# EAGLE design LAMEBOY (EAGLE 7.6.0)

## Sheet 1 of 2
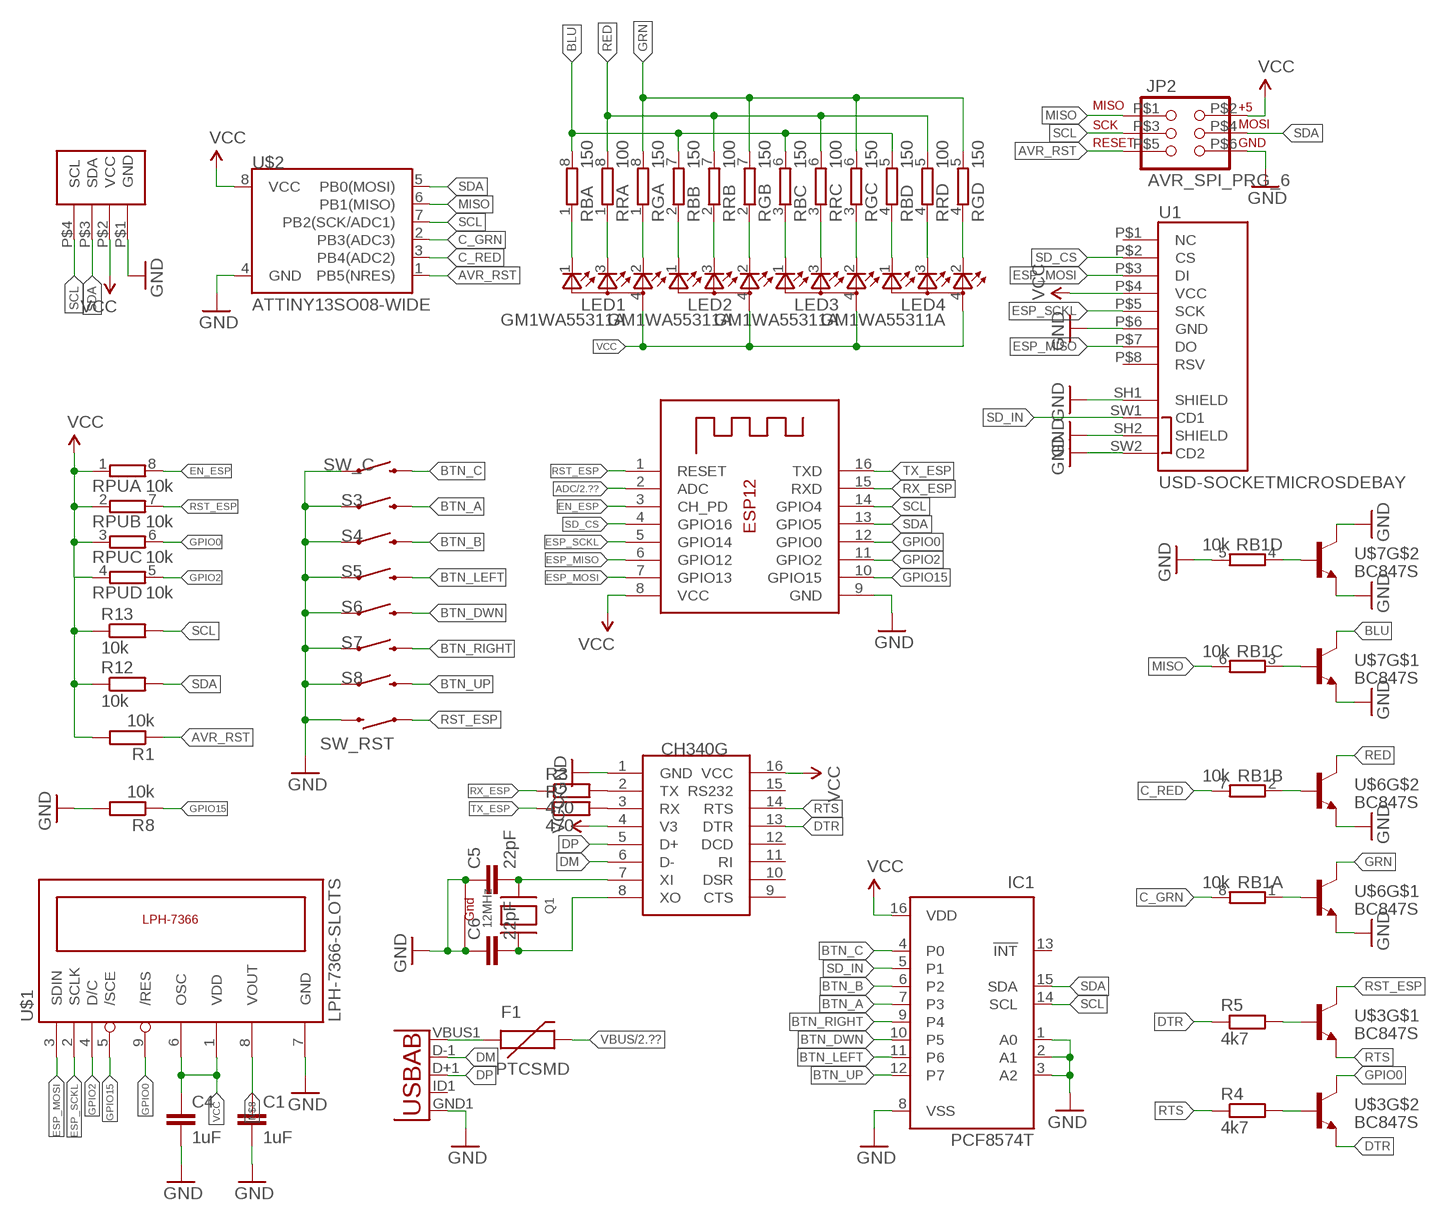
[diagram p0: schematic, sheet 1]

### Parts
C1  1uF  C-EUC0603K  [C0603K]
C4  1uF  C-EUC0603K  [C0603K]
C5  22pF  C-EUC0603K  [C0603K]
C6  22pF  C-EUC0603K  [C0603K]
CH340G  CH340GCH340G  [SOIC16]
F1  PTCSMD  [PTC-1206]
IC1  PCF8574T  [SO16W]
JP2  AVR_SPI_PRG_6  [2X3_SMD_PAD]
LED1  GM1WA55311A  [GM1WA55311A]
LED2  GM1WA55311A  [GM1WA55311A]
LED3  GM1WA55311A  [GM1WA55311A]
LED4  GM1WA55311A  [GM1WA55311A]
Q1  12MHz  XTAL-4-3225  [NX3225]
R1  10k  R-EU_R0603  [R0603]
R2  470  R-EU_R0603  [R0603]
R3  470  R-EU_R0603  [R0603]
R4  4k7  R-EU_R0603  [R0603]
R5  4k7  R-EU_R0603  [R0603]
R8  10k  R-EU_R0603  [R0603]
R12  10k  R-EU_R0603  [R0603]
R13  10k  R-EU_R0603  [R0603]
RB  150  4R-N0603-ARC  [0603-ARC]
RB1  10k  4R-N0603-ARC  [0603-ARC]
RG  150  4R-N0603-ARC  [0603-ARC]
RPU  10k  4R-N0603-ARC  [0603-ARC]
RR  100  4R-N0603-ARC  [0603-ARC]
S3  SWITCH-MOMENTARY-2SMD-4  [TACTILE_SWITCH_TALL]
S4  SWITCH-MOMENTARY-2SMD-4  [TACTILE_SWITCH_TALL]
S5  SWITCH-MOMENTARY-2SMD-4  [TACTILE_SWITCH_TALL]
S6  SWITCH-MOMENTARY-2SMD-4  [TACTILE_SWITCH_TALL]
S7  SWITCH-MOMENTARY-2SMD-4  [TACTILE_SWITCH_TALL]
S8  SWITCH-MOMENTARY-2SMD-4  [TACTILE_SWITCH_TALL]
SW_C  SWITCH-MOMENTARY-2-SMD-1101NE  [TACTILE-SWITCH-1101NE]
SW_RST  SWITCH-MOMENTARY-2-SMD-1101NE  [TACTILE-SWITCH-1101NE]
U1  USD-SOCKETMICROSDEBAY  [MICRO-SD-SOCKET-EBAY]
U2  USB  USB-ABCONN-11794  [USB-AB-MICRO-SMD_V03]
U$1  LPH-7366-SLOTS  [LPH-7366-SLOTS]
U$2  ATTINY13SO08-WIDE  [SO08-EIAJ]
U$3  BC847S  MMDT3904  [SOT363]
U$6  BC847S  MMDT3904  [SOT363]
U$7  BC847S  MMDT3904  [SOT363]
U$10  I2C_GROVE  [I2C_GROVE]
X1  ESP-12  [ESP-12]

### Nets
ADC: X1.2(ADC) ; also sheet 2
AVR_RST: JP2.P$5 R1.1 U$2.1(PB5(NRES))
BLU: RB.5 RB.6 RB.7 RB.8 U$7.3(C)
BTN_A: IC1.7(P3) S3.B2
BTN_B: IC1.6(P2) S4.B2
BTN_C: IC1.4(P0) SW_C.P$2
BTN_DWN: IC1.10(P5) S6.B2
BTN_LEFT: IC1.11(P6) S5.B2
BTN_RIGHT: IC1.9(P4) S7.B2
BTN_UP: IC1.12(P7) S8.B2
C_GRN: RB1.8 U$2.2(PB3(ADC3))
C_RED: RB1.7 U$2.3(PB4(ADC2))
DM: CH340G.6(D-) U2.D-1(D-)
DP: CH340G.5(D+) U2.D+1(D+)
DTR: CH340G.13(DTR) R5.1 U$3.1(E)
EN_ESP: RPU.8 X1.3(CH_PD)
ESP_MISO: U1.P$7(DO) X1.6(GPIO12)
ESP_MOSI: U1.P$3(DI) U$1.3(SDIN) X1.7(GPIO13)
ESP_SCKL: U1.P$5(SCK) U$1.2(SCLK) X1.5(GPIO14)
GND: C1.2 C4.2 C5.1 C6.1 CH340G.1(GND) IC1.1(A0) IC1.2(A1) IC1.3(A2) IC1.8(VSS) JP2.P$6 Q1.2(G2) Q1.4(G1) R8.2 RB1.5 S3.A2 S4.A2 S5.A2 S6.A2 S7.A2 S8.A2 SW_C.P$1 SW_RST.P$2 U1.P$6(GND) U1.SH1(SHIELD) U1.SH2(SHIELD) U1.SW2(CD2) U2.GND1(GND) U$1.7(GND) U$2.4(GND) U$6.1(E) U$6.4(E) U$7.1(E) U$7.4(E) U$7.6(C) U$10.P$1(GND) X1.9(GND) ; also sheet 2
GPIO0: RPU.6 U$1.9(/RES) U$3.6(C) X1.12(GPIO0)
GPIO2: RPU.5 U$1.4(D/C) X1.11(GPIO2)
GPIO15: R8.1 U$1.5(/SCE) X1.10(GPIO15)
GRN: RG.5 RG.6 RG.7 RG.8 U$6.3(C)
L2_R: LED1.3(CBLUE) RR.1
L3_B: LED1.1(CGREEN) RB.1
L4_G: LED1.2(CRED) RG.1
MISO: JP2.P$1 RB1.6 U$2.6(PB1(MISO))
N$1: LED4.1(CGREEN) RB.4
N$2: LED4.3(CBLUE) RR.4
N$3: LED4.2(CRED) RG.4
N$4: LED3.1(CGREEN) RB.3
N$5: LED3.3(CBLUE) RR.3
N$6: LED3.2(CRED) RG.3
N$7: LED2.1(CGREEN) RB.2
N$8: C1.1 U$1.8(VOUT)
N$9: LED2.3(CBLUE) RR.2
N$10: LED2.2(CRED) RG.2
N$11: RB1.1 U$6.5(B)
N$13: RB1.2 U$6.2(B)
N$17: C5.2 CH340G.7(XI) Q1.1(X1)
N$18: RB1.3 U$7.5(B)
N$19: RB1.4 U$7.2(B)
N$24: C6.2 CH340G.8(XO) Q1.3(X2)
N$25: R5.2 U$3.5(B)
N$26: CH340G.3(RX) R2.2
N$27: CH340G.2(TX) R3.2
N$28: R4.2 U$3.2(B)
RED: RR.5 RR.6 RR.7 RR.8 U$6.6(C)
RST_ESP: RPU.7 SW_RST.P$1 U$3.3(C) X1.1(RESET)
RTS: CH340G.14(RTS) R4.1 U$3.4(E)
RX_ESP: R3.1 X1.15(RXD)
SCL: IC1.14(SCL) JP2.P$3 R13.2 U$2.7(PB2(SCK/ADC1)) U$10.P$4(SCL) X1.14(GPIO4)
SD_CS: U1.P$2(CS) X1.4(GPIO16)
SD_IN: IC1.5(P1) U1.SW1(CD1)
SDA: IC1.15(SDA) JP2.P$4 R12.2 U$2.5(PB0(MOSI)) U$10.P$3(SDA) X1.13(GPIO5)
TX_ESP: R2.1 X1.16(TXD)
VBUS: F1.2 ; also sheet 2
VCC: C4.1 CH340G.4(V3) CH340G.16(VCC) IC1.16(VDD) JP2.P$2 LED1.4(A) LED2.4(A) LED3.4(A) LED4.4(A) R1.2 R12.1 R13.1 RPU.1 RPU.2 RPU.3 RPU.4 U1.P$4(VCC) U$1.1(VDD) U$1.6(OSC) U$2.8(VCC) U$10.P$2(VCC) X1.8(VCC) ; also sheet 2
VUSB: F1.1 U2.VBUS1(VBUS)
Unconnected: CH340G.9(CTS) CH340G.10(DSR) CH340G.11(RI) CH340G.12(DCD) CH340G.15(RS232) IC1.13(!INT) U1.P$1(NC) U1.P$8(RSV) U2.ID1(USBID)

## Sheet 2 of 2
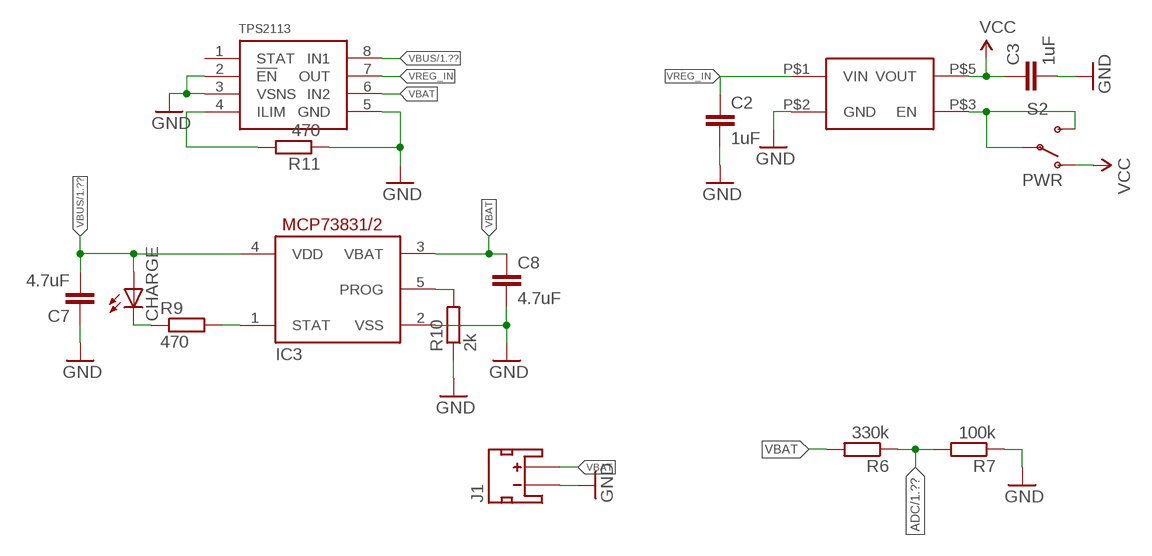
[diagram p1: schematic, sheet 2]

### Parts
C2  1uF  C-EUC0603K  [C0603K]
C3  1uF  C-EUC0603K  [C0603K]
C7  4.7uF  C-EUC0603K  [C0603K]
C8  4.7uF  C-EUC0603K  [C0603K]
CHARGE  LEDCHIP-LED0805  [CHIP-LED0805]
IC3  MCP73831  MCP73831/OT  [SOT23-5L]
J1  JST_2MM_MALE  [JST-2-SMD]
R6  330k  R-EU_R0603  [R0603]
R7  100k  R-EU_R0603  [R0603]
R9  470  R-EU_R0603  [R0603]
R10  2k  R-EU_R0603  [R0603]
R11  470  R-EU_R0603  [R0603]
S2  PWR  SWITCH-SPDT-SMD-A  [SWITCH-SPST-SMD-A]
U$4  TPS2113-PW  [TEXAS-PW]
U$9  AP2112KAP2112K  [AP2112]

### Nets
ADC: R6.1 R7.2 ; also sheet 1
GND: C2.2 C3.2 C7.1 C8.2 IC3.2(VSS) J1.1(-) R7.1 R10.1 R11.1 U$4.2(!EN) U$4.3(VSNS) U$4.5(GND) U$9.P$2(GND) ; also sheet 1
N$12: IC3.1(STAT) R9.2
N$15: CHARGE.C R9.1
N$20: R11.2 U$4.4(ILIM)
N$21: IC3.5(PROG) R10.2
VBAT: C8.1 IC3.3(VBAT) J1.2(+) R6.2 U$4.6(IN2)
VBUS: C7.2 CHARGE.A IC3.4(VDD) U$4.8(IN1) ; also sheet 1
VCC: C3.1 S2.1(O) U$9.P$5(VOUT) ; also sheet 1
VREG_IN: C2.1 U$4.7(OUT) U$9.P$1(VIN)
VREG_OUT: S2.2(P) S2.3(S) U$9.P$3(EN)
Unconnected: J1.NC1(PAD1) J1.NC2(PAD2) U$4.1(STAT)

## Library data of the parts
C1-C8 = rcl:C-EU: CAPACITOR, European symbol
CH340G = ch340g:CH340G: USB to TTL RS232 converter
CHARGE = led:LED: LED
F1 = SparkFun-PowerIC:PTC: Resettable Fuse PTC; PROD_ID: RES-11150
IC1 = micro-philips:PCF8574: I2C-Bus Remote 8-bit I/O expander http://www.semiconductors.philips.com/acrobat_download/datasheets/PCF8574_4.pdf; MPN: PCF8574T/3,512; OC_FARNELL: 1201255; OC_NEWARK: 70R6870
IC3 = adafruit:MCP73831: MCP73831/2 Miniature Single-Cell, Fully Integrated Li-Ion, Li-Polymer Charge Management Controllers. Nice and small simple lipoly charge controller, with adjustable current and status output (LED) http://www.ladyada.net/library/pcb/eaglelibrary.html
J1 = SparkFun-Connectors:JST_2MM_MALE: Mates to single-cell LiPo batteries. CONN-08352; PROD_ID: CONN-08352
JP2 = SparkFun-Connectors:AVR_SPI_PRG_6: AVR ISP 6 Pin This is the reduced ISP connector for AVR programming. Common on Arduino. This footprint will take up less PCB space and can be used with a 10-pin to 6-pin adapter such as SKU: BOB-08508 **Special note about "TEST_POINT" package. The stop mask is on the top side, so if you want your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
LED1-LED4 = led:GM1WA55311A: Chip LED RGB Source: http://document.sharpsma.com/files/GM1WA55311A_SS.pdf
Q1 = adafruit:XTAL-4: Classic 4-pin 3.2 x 2.5mm crystal
R1-R13 = rcl:R-EU_: RESISTOR, European symbol
RB RB1 RG RPU RR = resistor-dil:4R-N: Array Chip Resistor Source: RS Component / Phycomp; OC_FARNELL: unknown; OC_NEWARK: unknown
S2 = SparkFun-Electromechanical:SWITCH-SPDT: SPDT Switch Simple slide switch, Spark Fun Electronics SKU : COM-00102 DPDT SMT slide switch, AYZ0202, SWCH-08179
S3-S8 = SparkFun-Electromechanical:SWITCH-MOMENTARY-2: Various NO switches- pushbuttons, reed, etc; PROD_ID: SWCH-11966
SW_C SW_RST = SparkFun-Electromechanical:SWITCH-MOMENTARY-2: Various NO switches- pushbuttons, reed, etc
U1 = SparkFun-Connectors:USD-SOCKET: microSD Socket Push-push type uSD socket. Schematic element and footprint production proven. Spark Fun Electronics SKU : PRT-00127. tDoc lines correctly indicate media card edge positions when inserting (unlocked, locked, depressed). NOTE: CD1 and CD2 are connected internally
U2 = SparkFun-Connectors:USB-AB: This is a USB AB connector that is compatible with USB OTG. i.e. this connector can serve as a host or device; PROD_ID: CONN-11794
U$1 = lph-7366:LPH-7366-SLOTS
U$2 = SparkFun-DigitalIC:ATTINY13: Atmel 8-pin 1kB flash uC
U$3 U$6 U$7 = SparkFun-DiscreteSemi:MMDT3904: Dual NPN transistor
U$4 = TPS2113:TPS2113-PW
U$9 = TPS2113:AP2112K
U$10 = TPS2113:I2C_GROVE
X1 = adafruit:ESP-12

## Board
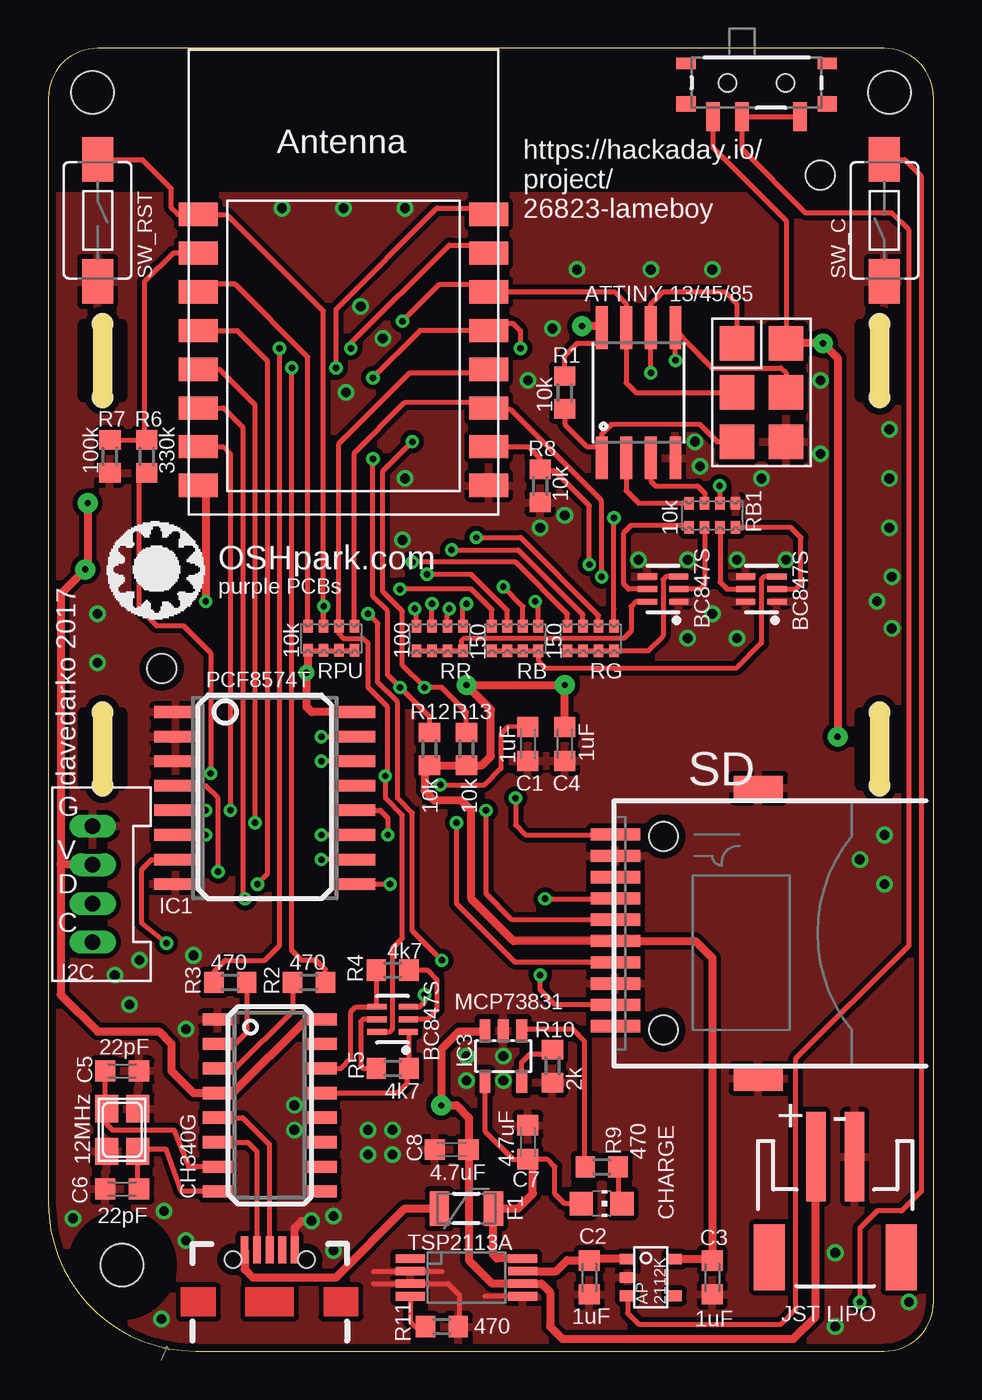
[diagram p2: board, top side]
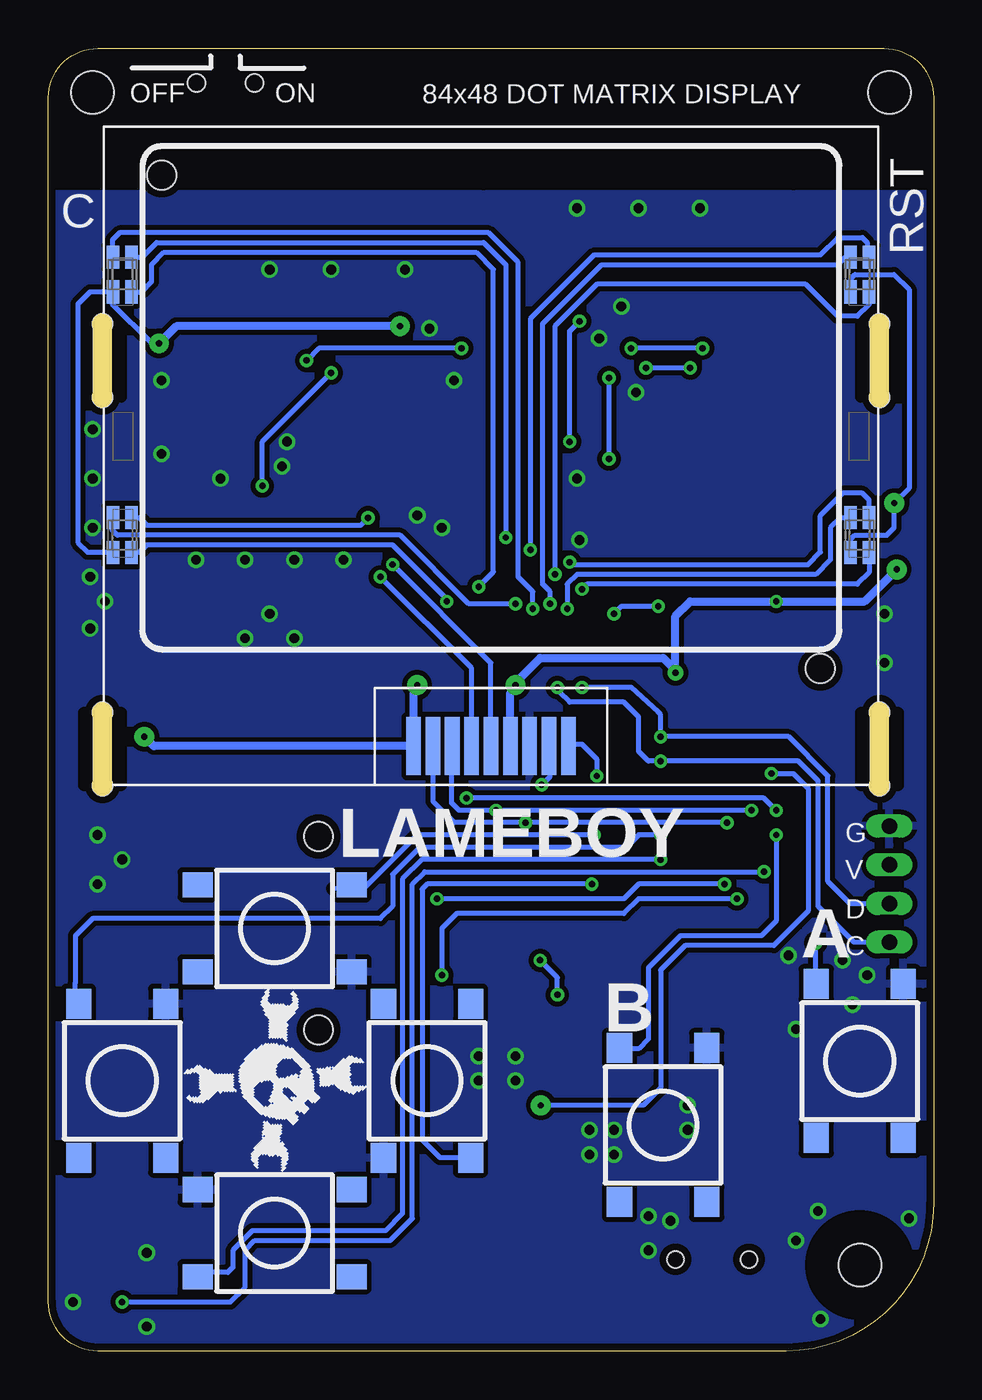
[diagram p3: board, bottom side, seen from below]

Size 45.72 x 67.31 mm. Coordinates in mm from the lower left corner, seen from the top.
Outline: 0,64.77 0,7.62 arc90 7.62,0 43.18,0 arc90 45.72,2.54 45.72,64.77 arc90 43.18,67.31 2.54,67.31 arc90 0,64.77
Copper layers (1*16): Top 0.0356mm / dielectric 1.5011mm / Bottom 0.0356mm
Design rules "LaenPCBOrder *": minimum track width 6mil, minimum drill 13mil, track to track 6mil, track to pad 6mil, pad to pad 6mil, via to via 6mil, smd to smd 6mil, copper to edge 15mil, drill to drill 6mil, minimum pad ring 7mil, minimum via ring 7mil, stop-mask expansion 3mil, vias tented up to drill 200mil, thermal gap 10mil
Holes 2.2 mm at 3.81,4.45 2.29,65.02 43.43,65.02
tRestrict: area 1.3,1.9 to 6.3,6.9
bRestrict: area 1.3,1.9 to 6.3,6.9

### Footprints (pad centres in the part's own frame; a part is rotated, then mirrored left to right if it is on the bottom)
C0603K = smd 1.05 x 1.08: 1 -0.875,0; 2 0.875,0
SOIC16 = smd 0.635 x 1.524: 1 -4.445,-2.695; 2 -3.175,-2.695; 3 -1.905,-2.695; 4 -0.635,-2.695; 5 0.635,-2.695; 6 1.905,-2.695; 7 3.175,-2.695; 8 4.445,-2.695; 9 4.445,2.695; 10 3.175,2.695; 11 1.905,2.695; 12 0.635,2.695; 13 -0.635,2.695; 14 -1.905,2.695; 15 -3.175,2.695; 16 -4.445,2.695
CHIP-LED0805 = smd 1.2 x 1.2: A 0,-1.05; C 0,1.05
PTC-1206 = smd 1 x 1.8: 1 -1.4,0; 2 1.4,0
SO16W = smd 0.6 x 2.2: 1 -4.445,-4.6; 2 -3.175,-4.6; 3 -1.905,-4.6; 4 -0.635,-4.6; 5 0.635,-4.6; 6 1.905,-4.6; 7 3.175,-4.6; 8 4.445,-4.6; 9 4.445,4.6; 10 3.175,4.6; 11 1.905,4.6; 12 0.635,4.6; 13 -0.635,4.6; 14 -1.905,4.6; 15 -3.175,4.6; 16 -4.445,4.6
SOT23-5L = smd 0.55 x 1.2: 1 -0.95,-1.3; 2 0,-1.3; 3 0.95,-1.3; 4 0.95,1.3; 5 -0.95,1.3
JST-2-SMD = smd 1 x 4.6: 1 -1,-3.7; 2 1,-3.7 | smd 1.6 x 3.4: NC1 -3.4,1.5; NC2 3.4,1.5
2X3_SMD_PAD = smd 1.778 x 1.778: P$1 -1.27,2.54; P$2 1.27,2.54; P$3 -1.27,0; P$4 1.27,0; P$5 -1.27,-2.54; P$6 1.27,-2.54
GM1WA55311A = smd 0.65 x 1.2: 1 -0.475,0.9; 2 -0.475,-0.9; 3 0.475,-0.9; 4 0.475,0.9
NX3225 = smd 1.4 x 1.2: 1 -1.1,-0.8; 2 1.1,-0.8; 3 1.1,0.8; 4 -1.1,0.8
R0603 = smd 1 x 1.1: 1 -0.85,0; 2 0.85,0
0603-ARC = smd 0.5 x 0.65: 1 -1.2,-0.625; 2 -0.4,-0.625; 3 0.4,-0.625; 4 1.2,-0.625; 5 1.2,0.625; 6 0.4,0.625; 7 -0.4,0.625; 8 -1.2,0.625
SWITCH-SPST-SMD-A = smd 0.7 x 1.5: 1 -2.25,-1.75; 2 -0.75,-1.75; 3 2.25,-1.75 | smd 1 x 0.6: GND1 -3.65,1; GND3 3.65,1 | smd 1 x 0.8: GND2 -3.65,-1.1; GND4 3.65,-1.1 | hole 0.9: -1.5,0; 1.5,0
TACTILE_SWITCH_TALL = smd 1.55 x 1.3: A1 -3.975,-2.25; A2 3.975,-2.25; B1 -3.975,2.25; B2 3.975,2.25
TACTILE-SWITCH-1101NE = smd 2.3 x 1.6: P$1 -3.15,0; P$2 3.15,0
MICRO-SD-SOCKET-EBAY = smd 0.63 x 2.54: P$1 -2.9,-5; P$2 -1.8,-5; P$4 0.4,-5; P$5 1.5,-5; P$6 2.6,-5; P$7 3.7,-5; P$8 4.8,-5; SW1 -5.1,-5; SW2 -4,-5 | smd 0.635 x 2.54: P$3 -0.7,-5 | smd 1.27 x 2.54: SH1 -7.5,2.37; SH2 7.5,2.37 | hole 1.5: -5,-2.52; 5,-2.52
USB-AB-MICRO-SMD_V03 = smd 1.4 x 0.4: D+1 2.7,0; D-1 2.7,0.65; GND1 2.7,-1.3; ID1 2.7,-0.65; VBUS1 2.7,1.3 | hole 0.85: 2.2,1.9; 2.2,-1.9
LPH-7366-SLOTS = smd 0.75 x 3: 1 4,17; 2 3,17; 3 2,17; 4 1,17; 5 0,17; 6 -1,17; 7 -2,17; 8 -3,17; 9 -4,17 | hole 1.5: -17,13; 17,-12.5 | hole 1.016: -20.066,19.05; -20.066,15.24; 20.066,19.05; 20.066,15.24; 20.066,-1.016; 20.066,-4.826; -20.066,-1.016; -20.066,-4.826
SO08-EIAJ = smd 0.61 x 2.21: 1 -1.905,-3.378; 2 -0.635,-3.378; 3 0.635,-3.378; 4 1.905,-3.378; 5 1.905,3.353; 6 0.635,3.353; 7 -0.635,3.353; 8 -1.905,3.353
SOT363 = smd 0.3 x 0.99: 1 -0.65,-0.8; 2 0,-0.8; 3 0.65,-0.8; 4 0.65,0.81; 5 0,0.81; 6 -0.65,0.81
TEXAS-PW = smd 1.5 x 0.45: 1 -2.9,0.975; 2 -2.9,0.325; 3 -2.9,-0.325; 4 -2.9,-0.975; 5 2.9,-0.975; 6 2.9,-0.325; 7 2.9,0.325; 8 2.9,0.975
AP2112 = smd 0.55 x 0.8: P$1 0.95,1.2; P$2 0,1.2; P$3 -0.95,1.2; P$4 -0.95,-1.2; P$5 0.95,-1.2
I2C_GROVE = drill 0.8 long: P$1 0,3; P$2 0,1; P$3 0,-1; P$4 0,-3
ESP-12 = smd 2 x 1.2: 1 -7.5,4.5; 2 -7.5,2.5; 3 -7.5,0.5; 4 -7.5,-1.5; 5 -7.5,-3.5; 6 -7.5,-5.5; 7 -7.5,-7.5; 8 -7.5,-9.5; 9 7.5,-9.5; 10 7.5,-7.5; 11 7.5,-5.5; 12 7.5,-3.5; 13 7.5,-1.5; 14 7.5,0.5; 15 7.5,2.5; 16 7.5,4.5

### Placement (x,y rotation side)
C1  24.77,31.37 270 top
C2  27.94,3.81 270 top
C3  34.29,3.81 270 top
C4  26.67,31.37 270 top
C5  3.81,14.48 180 top
C6  3.81,8.38 0 top
C7  24.77,10.79 270 top
C8  20.83,10.41 180 top
CH340G  11.43,12.7 270 top
CHARGE  28.57,7.62 270 top
F1  21.59,7.37 0 top
IC1  11.18,28.57 270 top
IC3  23.5,15.24 180 top
J1  40.64,6.35 180 top
JP2  36.83,49.53 0 top
LED1  41.91,42.16 180 bottom
LED2  41.91,55.63 180 bottom
LED3  3.81,55.63 180 bottom
LED4  3.81,42.16 180 bottom
Q1  3.81,11.43 270 top
R1  26.67,49.53 90 top
R2  13.46,19.05 180 top
R3  9.4,19.05 0 top
R4  17.78,19.68 0 top
R5  17.78,14.61 180 top
R6  5.08,46.23 270 top
R7  3.17,46.23 90 top
R8  25.4,44.7 270 top
R9  28.57,9.53 180 top
R10  26.04,14.73 90 top
R11  20.32,1.27 180 top
R12  19.68,31.11 90 top
R13  21.59,31.11 90 top
RB  24.1,36.82 180 top
RB1  34.29,43.18 0 top
RG  28.01,36.82 180 top
RPU  14.61,36.83 0 top
RR  20.21,36.82 180 top
S2  36.58,65.53 0 top
S3  3.81,14.99 90 bottom
S4  13.97,11.68 90 bottom
S5  41.91,13.97 90 bottom
S6  34.04,6.1 180 bottom
S7  26.16,13.97 270 bottom
S8  34.04,21.84 0 bottom
SW_C  43.18,58.42 90 top
SW_RST  2.54,58.42 270 top
U1  34.29,21.59 270 top
U2  11.43,2.54 90 top
U$1  22.86,48.26 180 bottom
U$2  30.48,49.53 0 top
U$3  17.78,17.14 90 top
U$4  21.59,3.81 0 top
U$5  [OSHPARK_LOGO]  14.48,40.39 0 top
U$6  31.75,39.37 90 top
U$7  36.83,39.37 90 top
U$8  [HACKADAY_LOGO]  33.79,13.73 45 bottom
U$9  31.11,3.81 90 top
U$10  2.29,24.13 0 top
X1  15.24,54.23 0 top

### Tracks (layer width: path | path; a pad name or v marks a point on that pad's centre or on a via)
ADC
  Top 0.254: 7.66,57.19 X1.2 6.44,56.73 4.95,55.24 4.95,47.2 R6.1 R7.2
AVR_RST
  Top 0.254: R1.1 26.67,47.88 27.81,46.74 28.37,46.74 U$2.1 28.57,47.37 29.08,47.88 33.66,47.88 34.54,46.99 JP2.P$5
BLU
  Top 0.254: RB.5 RB.6 RB.7 RB.8 25.3,35.66 25.65,35.31 35.56,35.31 36.83,36.58 36.83,39.88 36.97,40.02 U$7.3
BTN_A  (via drill 0.33)
  Top 0.254: v6.1,21.08 4.83,22.1 4.83,24.89 5.33,25.4 IC1.7
  Bottom 0.254: S3.B2 6.1,19.25 v6.1,21.08
BTN_B  (via drill 0.33)
  Top 0.254: IC1.6 v8.13,26.67
  Bottom 0.254: v8.13,26.67 8.13,22.23 8.89,21.46 13.08,21.46 14.73,19.81 14.73,16.13 15.24,15.62 16.05,15.62 S4.B2
BTN_C  (via drill 0.33)
  Top 0.254: SW_C.P$2 44.22,61.57 45.09,60.71 45.09,8.26 44.07,7.24 42.8,7.24 41.91,6.35 v41.91,2.54 | v8.76,24.77 8.76,28.57 8.13,29.21 IC1.4
  Bottom 0.254: v41.91,2.54 36.32,2.54 35.56,3.3 35.56,5.21 35.05,5.71 28.07,5.71 26.92,6.86 26.92,24.13 26.29,24.77 v8.76,24.77
BTN_DWN  (via drill 0.33)
  Top 0.254: IC1.10 v14.1,25.4
  Bottom 0.254: v14.1,25.4 26.42,25.4 27.43,24.38 27.43,7.11 28.32,6.22 35.18,6.22 36.2,5.21 36.2,4.32 36.45,4.06 37.52,4.06 37.55,4.1 S6.B2
BTN_LEFT  (via drill 0.33)
  Top 0.254: IC1.11 v14.1,26.67
  Bottom 0.254: v14.1,26.67 15.24,26.67 15.88,26.04 26.54,26.04 27.94,24.64 27.94,22.99 28.57,22.35 43.43,22.35 44.32,21.46 44.32,19.05 44.32,18.11 | 44.32,18.11 44.32,17.37 | S5.B2 44.32,18.11
BTN_RIGHT  (via drill 0.33)
  Top 0.254: IC1.9 v17.65,24.13
  Bottom 0.254: v17.65,24.13 26.16,24.13 26.42,23.88 26.42,10.92 25.49,9.99 S7.B2
BTN_UP  (via drill 0.33)
  Top 0.254: IC1.12 17.14,27.94 17.53,27.56 v17.53,26.67
  Bottom 0.254: v17.53,26.67 26.67,26.67 29.46,23.88 30.48,23.89 | 30.48,23.89 30.99,23.9 | S8.B2 30.37,23.89 30.48,23.89
C_GRN
  Top 0.254: U$2.2 29.84,44.45 30.48,43.81 31.81,43.81 RB1.8
C_RED
  Top 0.254: U$2.3 31.11,44.96 31.37,44.7 33.53,44.7 33.91,44.32 33.91,43.82 RB1.7
DM
  Top 0.254: CH340G.6 10.29,10.79 10.78,10.3 U2.D-1
DP
  Top 0.254: CH340G.5 10.03,12.06 11.43,10.67 U2.D+1
DTR
  Top 0.254: U$3.1 18.63,16.45 R5.1 18.54,14.52 18.54,13.84 18.03,13.34 CH340G.13
EN_ESP
  Top 0.254: RPU.8 13.4,51.37 9.65,55.12 7.75,55.12 X1.3
ESP_MISO  (via drill 0.33)
  Top 0.254: X1.6 9.06,48.73 10.03,47.75 10.03,23.5 v10.16,23.37 | U1.P$7 26.18,17.89 25.4,18.67 v25.4,19.43
  Bottom 0.254: v10.16,23.37 15.24,23.37 16,22.61 24.64,22.61 25.4,21.84 v25.4,19.43
ESP_MOSI  (via drill 0.33, 0.33 pad 0.61)
  Top 0.254: X1.7 9.02,46.73 9.4,46.35 v9.4,27.94 | U1.P$3 23.94,22.29 22.61,23.62 v22.61,27.94
  Bottom 0.254: v9.4,27.94 v22.61,27.94 24.51,27.94 24.89,28.32 24.89,31.23 U$1.3
ESP_SCKL  (via drill 0.33, 0.33 pad 0.61)
  Top 0.254: X1.5 8.83,50.73 10.67,48.9 v10.67,27.3 | v21.08,27.3 21.08,23.11 24.11,20.09 U1.P$5
  Bottom 0.254: v10.67,27.3 v21.08,27.3 24.77,27.3 25.86,28.4 U$1.2
GND  (via drill 0.5)
  Top 0.254: U$4.3 18.74,3.48 | 18.74,3.48 20.64,3.48 21.21,2.92 21.21,1.31 R11.1 | 16.79,4.12 18.37,4.12 | 18.37,4.12 18.74,4.12 | 18.37,4.12 20.33,4.12 | 16.79,3.48 18.74,3.48 | 22.55,2.85 24.45,2.85
  Top 0.406: U2.GND1 12.73,6.38 13.08,6.73 v13.59,6.73
  other vias: 1.27,6.86 5.84,1.65 40.64,1.27 40.64,5.08 44.45,2.54 33.02,40.89 30.48,40.89 35.56,40.89 38.1,40.89 34.29,38.1 33.02,36.83 35.56,36.83 2.54,35.56 2.54,38.1 33.4,46.99 33.66,45.72 36.83,45.09 43.43,47.62 43.43,45.09 42.8,38.73 43.56,40.01 43.43,42.55 43.56,37.34 26.67,43.18 25.4,42.55 18.41,45.09 18.29,41.91 39.88,46.35 34.29,55.88 31.11,55.88 27.3,55.88 12.06,59.05 15.24,59.05 18.41,59.05 39.88,50.16 24.77,50.16 26.04,52.83 16.13,53.98 15.37,49.53 17.27,52.32 21.59,15.24 21.59,13.97 23.5,15.24 23.5,13.97 43.18,26.67 41.91,25.4 43.18,24.13 17.78,11.43 17.78,10.16 14.73,6.99 14.73,5.21 16.51,11.43 16.51,10.16 12.7,12.7 12.7,11.43 4.7,20.19 3.43,19.43 4.19,17.91 7.49,20.45 7.11,16.64 5.97,7.24 7.11,5.71
  pour Bottom (isolate 0.254): -2.54,59.77 48.26,59.77 48.26,-5.08 -2.54,-5.08
  pour Top (isolate 0.254): -3.81,59.69 49.53,59.69 49.53,-2.54 -3.81,-2.54
GPIO0  (via drill 0.33 pad 0.61)
  Top 0.254: X1.12 22.56,50.55 18.67,50.55 15.01,46.88 RPU.6 15.01,37.06 15.24,36.83 16.26,36.83 16.51,36.58 16.51,34.29 17.53,33.27 17.53,29.59 v17.4,29.72 17.4,28.57 18.29,27.69 18.29,21.34 17.78,20.83 17.78,16.64 17.64,16.5 U$3.6
  Bottom 0.254: U$1.9 18.86,31.3 18.8,31.37 18.16,31.37 17.4,30.61 v17.4,29.72
GPIO2  (via drill 0.33 pad 0.61)
  Top 0.254: RPU.5 15.8,46.41 18.41,49.02 22.91,49.02 X1.11 23.16,48.64 23.88,48.64 28.57,43.94 v28.57,40.01
  Bottom 0.254: U$1.4 23.86,35.29 v28.57,40.01
GPIO15  (via drill 0.33 pad 0.61)
  Top 0.254: v27.94,40.64 27.94,43.69 26.16,45.47 25.49,45.47 R8.1 25.4,46.1 24.77,46.73 X1.10
  Top 0.406: 25.18,45.84 R8.1
  Bottom 0.254: U$1.5 22.86,35.56 v27.94,40.64
GRN
  Top 0.254: RG.5 RG.6 RG.7 RG.8 30.98,36.19 31.75,36.96 31.75,39.88 31.89,40.02 U$6.3
L2_R  (via drill 0.33 pad 0.64)
  Top 0.254: RR.1 21.41,38.56 v21.59,38.61
  Bottom 0.254: v21.59,38.61 24,38.61 27.56,42.16 42.16,42.16 42.42,42.42 42.42,43.09 LED1.3
L3_B  (via drill 0.33 pad 0.64)
  Top 0.254: RB.1 25.3,38.58 v25.15,38.73
  Bottom 0.254: v25.15,38.73 25.15,38.86 27.94,41.66 40.64,41.66 41.03,41.26 LED1.1
L4_G  (via drill 0.33 pad 0.64)
  Top 0.254: RG.1 29.21,38.36 v29.21,43.05
  Bottom 0.254: LED1.2 41.03,43.06 40.64,42.67 29.59,42.67 v29.21,43.05
MISO  (via drill 0.33)
  Top 0.254: 31.11,52.7 U$2.6 | U$2.6 31.11,54.1 31.75,54.74 34.92,54.74 35.56,54.1 JP2.P$1 | RB1.6 34.69,44.69 v34.67,44.7 | v31.11,50.55 U$2.6
  Bottom 0.254: v34.67,44.7 34.67,46.99 v31.11,50.55
N$1  (via drill 0.33 pad 0.64)
  Top 0.254: RB.4 22.9,38.31 21.84,39.37 v18.16,39.37
  Bottom 0.254: LED4.1 3.34,40.23 3.94,39.62 17.91,39.62 v18.16,39.37
N$2  (via drill 0.33 pad 0.64)
  Top 0.254: RR.4 19.01,38.27 v18.92,38.35
  Bottom 0.254: LED4.3 4.83,43.05 5.33,42.55 5.33,40.89 6.1,40.13 18.41,40.13 18.92,39.62 v18.92,38.35
N$3  (via drill 0.33 pad 0.64)
  Top 0.254: RG.4 26.81,38.09 24.13,40.77 v18.8,40.77
  Bottom 0.254: v18.8,40.77 18.67,40.64 6.48,40.64 5.84,41.27 5.84,43.18 4.7,44.32 3.68,44.32 3.34,43.98 LED4.2
N$4  (via drill 0.33 pad 0.64)
  Top 0.254: RB.3 23.7,38.27 21.84,40.13 v19.56,40.13
  Bottom 0.254: LED3.1 3.34,54.07 3.94,53.47 4.95,53.47 6.6,55.12 17.4,55.12 19.56,52.96 v19.56,40.13
N$5  (via drill 0.33 pad 0.64)
  Top 0.254: RR.3 v19.81,38.61
  Bottom 0.254: v19.81,38.61 19.81,39.24 20.19,39.62 20.19,53.09 17.14,56.13 4.95,56.13 4.57,56.52 4.3,56.52 LED3.3
N$6  (via drill 0.33 pad 0.64)
  Top 0.254: RG.3 27.61,38.05 24.26,41.4 v20.83,41.4
  Bottom 0.254: v20.83,41.4 20.83,53.34 17.53,56.64 5.84,56.64 4.95,57.53 3.68,57.53 3.43,57.28 3.43,56.62 LED3.2
N$7  (via drill 0.33 pad 0.64)
  Top 0.254: RB.2 24.5,38.47 v23.5,39.5
  Bottom 0.254: v23.5,39.5 22.73,40.26 22.73,55.88 23.62,56.77 39.75,56.77 40.39,56.13 40.39,55.24 40.91,54.73 LED2.1
N$8  (via drill 0.33 pad 0.61)
  Top 0.254: v20.24,29.26 22.53,29.26 23.37,30.1 23.37,31.88 23.75,32.26 C1.1
  Bottom 0.254: v20.24,29.26 19.81,29.69 19.81,30.99 U$1.8
N$9  (via drill 0.33 pad 0.64)
  Top 0.254: RR.2 20.61,38.19 v20.7,38.35
  Bottom 0.254: v20.7,38.35 20.7,39.24 21.46,40.01 21.46,56.26 22.99,57.78 42.04,57.78 42.42,57.4 42.42,56.56 LED2.3
N$10  (via drill 0.33 pad 0.64)
  Top 0.254: v22.1,42.04 24.38,42.04 28.41,38.02 RG.2
  Bottom 0.254: LED2.2 40.88,56.52 40.13,57.28 23.24,57.28 22.1,56.13 v22.1,42.04
N$11
  Top 0.254: U$6.5 29.97,39.37 29.72,39.62 29.72,42.29 30.1,42.67 32.97,42.67 RB1.1
N$12
  Top 0.254: IC3.1 24.45,16.57 24.51,16.64 27.05,16.64 27.69,16 27.69,9.56 R9.2
N$13
  Top 0.254: RB1.2 33.89,39.6 33.66,39.37 U$6.2
N$15
  Top 0.254: R9.1 29.43,7.82 CHARGE.C
N$17
  Top 0.254: CH340G.7 7.24,9.53 6.48,11.43 3.3,11.43 3.01,11.72 Q1.1 2.94,12.61 C5.2
N$18
  Top 0.254: RB1.3 34.69,39.73 35.05,39.37 U$7.5
N$19
  Top 0.254: U$7.2 38.61,39.37 38.86,39.62 38.86,42.04 38.35,42.55 RB1.4
N$20
  Top 0.254: U$4.4 18.69,1.5 18.92,1.27 R11.2
N$21
  Top 0.254: IC3.5 24.45,14.92 24.89,15.37 25.91,15.37 26.16,15.49 26.16,15.58 R10.2
N$24
  Top 0.254: CH340G.8 6.86,8.26 6.1,10.41 4.69,10.41 Q1.3 4.61,8.46 C6.2
N$25
  Top 0.254: U$3.5 16.26,17.14 16.13,17.02 16.13,14.73 16.26,14.61 R5.2
N$26
  Top 0.254: CH340G.3 9.65,14.61 12.61,17.57 R2.2
N$27
  Top 0.254: CH340G.2 9.65,15.88 10.25,16.47 R3.2
N$28
  Top 0.254: R4.2 19.56,19.68 20.07,19.18 20.07,17.65 19.56,17.14 U$3.2
RED
  Top 0.254: RR.5 RR.6 RR.7 RR.8 21.34,36.27 21.34,36.7 21.46,36.83 29.72,36.83 30.1,37.21 30.1,38.48 30.34,38.72 U$6.6
RST_ESP  (via drill 0.33, 0.33 pad 0.64)
  Top 0.254: v20.32,20.19 18.8,21.72 18.8,27.81 18.03,28.57 18.03,33.53 17.02,34.54 17.02,37.59 v16.51,38.1 | SW_RST.P$1 4.85,61.57 6.35,60.07 6.35,59.05 6.67,58.74 X1.1 9.22,58.73 14.21,53.74 RPU.7 14.22,37.44 v14.22,38.48 | U$3.3 19.19,17.8 19.43,18.03 v19.43,18.41
  Bottom 0.254: v19.43,18.41 19.43,19.3 v20.32,20.19 | v14.22,38.48 16.13,38.48 v16.51,38.1
RTS
  Top 0.254: R4.1 16.93,17.84 U$3.4 16.95,17.78 15.88,17.78 15.62,17.53 15.62,15.11 15.11,14.61 CH340G.14
RX_ESP  (via drill 0.33 pad 0.64)
  Top 0.254: v11.94,51.82 11.94,20.95 11.18,20.19 9.14,20.19 8.55,19.6 R3.1 | v15.62,51.82 15.62,52.07 20.7,57.15 22.7,57.15 X1.15
  Bottom 0.254: v11.94,51.82 v15.62,51.82
SCL  (via drill 0.33)
  Top 0.254: JP2.P$3 30.35,49.53 29.84,50.04 U$2.7 29.84,54.1 29.22,54.73 X1.14 22.73,55.12 20.19,55.12 v18.29,53.21 | v14.1,30.48 IC1.14 | v18.8,46.99 17.27,45.47 17.27,39.24 18.29,38.23 18.29,35.43 v19.43,34.29 20.32,34.29 21.59,33.02 R13.2
  Bottom 0.254: v19.43,34.29 19.3,34.04 18.8,33.53 16,33.53 15.24,32.77 15.24,30.99 14.73,30.48 v14.1,30.48 6.99,30.48 5.97,29.46 5.97,22.99 4.11,21.13 U$10.P$4 | v18.8,46.99 18.8,52.7 v18.29,53.21
SD_CS  (via drill 0.33)
  Top 0.254: X1.4 9.76,52.73 11.3,51.18 11.3,24.64 v10.79,24.13 | v25.65,23.37 29.27,23.37 U1.P$2
  Bottom 0.254: v10.79,24.13 15.24,24.13 16,23.37 v25.65,23.37
SD_IN  (via drill 0.33)
  Top 0.254: IC1.5 v8.13,27.94 | v24.13,28.57 24.13,27.18 24.64,26.67 29.27,26.67 U1.SW1
  Bottom 0.254: v8.13,27.94 8.76,28.57 v24.13,28.57
SDA  (via drill 0.33, 0.33 pad 0.64)
  Top 0.254: v32.38,51.18 U$2.5 32.94,52.15 34.29,50.8 37.85,50.8 38.1,50.55 JP2.P$4 | v14.1,31.75 IC1.15 | v16.76,46.1 16.76,38.99 17.53,38.23 17.53,34.92 v18.16,34.29 19.68,32.77 R12.2 | v16.76,50.29 19.2,52.73 X1.13 22.76,53.09 24,53.09 24.38,52.7 v24.38,51.82
  Bottom 0.254: v24.38,51.82 31.75,51.82 v32.38,51.18 | v18.16,34.29 15.62,34.29 14.22,33.02 14.1,32.89 v14.1,31.75 7.49,31.75 5.46,29.72 5.46,24.26 4.33,23.13 U$10.P$3 | v16.76,46.1 v16.76,50.29
TX_ESP  (via drill 0.33 pad 0.64)
  Top 0.254: v12.57,50.8 12.57,20.7 13.08,20.19 13.84,20.19 14.31,19.72 R2.1 | v14.86,50.8 14.86,53.85 20.07,59.05 22.68,59.05 X1.16
  Bottom 0.254: v12.57,50.8 v14.86,50.8
VBAT  (via drill 0.33 pad 0.61, 0.33 pad 1.02)
  Top 0.254: v8.38,29.84 8.38,36.07 6.99,37.47 5.59,37.47 4.7,38.35 4.7,44.96 5.08,45.34 R6.2
  Top 0.406: J1.2 39.62,11.3 39.62,1.78 38.48,0.64 26.54,0.64 25.91,1.27 25.91,3.05 25.47,3.48 U$4.6 22.93,3.48 21.72,4.7 C8.1 | 21.69,10.51 C8.1 | IC3.3 22.52,16.51 21.21,16.51 20.32,15.62 20.32,12.73 v20.29,12.7 21.08,12.7 21.72,12.06 21.72,10.43 C8.1
  Bottom 0.254: v8.38,29.84 7.24,29.84 6.48,29.08 6.48,22.73 8.26,20.95 12.83,20.95 14.1,19.68 14.1,13.59 14.99,12.7 v20.29,12.7
VBUS
  Top 0.254: IC3.4 22.55,11.36 24,9.91 24.77,9.9 C7.2 24.78,9.91 25.78,9.91 26.16,9.53 26.16,8.13 26.67,7.62 CHARGE.A
  Top 0.406: U$4.8 23.16,4.79 22.99,4.95 22.99,6.98 F1.2 24.26,7.37 25.02,8.13 25.02,9.78 C7.2
VCC  (via drill 0.33, 0.33 pad 0.81, 0.33 pad 1.02)
  Top 0.254: RPU.4 RPU.3 RPU.2 RPU.1 | R1.2 26.67,51.44 27.3,52.07 28.5,52.07 U$2.8 | 13.4,34.98 v13.34,35.05 | S2.1 34.33,62.19 38.1,58.42 JP2.P$2
  Top 0.406: CH340G.16 13.34,17.14 9.53,13.34 CH340G.4 7.49,13.34 6.35,14.48 6.35,15.88 5.71,16.51 2.54,16.51 0.64,18.41 0.64,25.15 | U$2.8 28.57,52.96 v27.56,52.96 | JP2.P$2 v40.01,52.07 40.77,51.31 v40.77,31.75 | v2.03,43.81 2.03,40.39 v1.91,40.39 0.64,39.12 0.64,25.15 | RPU.1 13.4,34.98 | IC1.16 13.59,33.02 13.34,33.27 v13.34,35.05 | X1.8 8.12,44.7 v8.13,38.73 | 40.64,31.88 v40.77,31.75 | C4.1 v26.67,34.42 v21.59,34.42 22.86,33.15 22.86,30.73 22.39,30.27 R13.1 R12.1 19.47,30.27 19.43,29.97 19.43,28.96 19.94,28.45 21.34,28.45 21.84,27.94 21.84,23.37 24.02,21.19 U1.P$4 33.42,21.19 34.29,20.32 C3.1 34.22,4.76 U$9.P$5 | 40.64,31.62 v40.77,31.75 | U$10.P$2 2.27,25.15 0.64,25.15
  Bottom 0.254: LED3.4 4.29,55.4 4.06,55.63 2.03,55.63 1.27,54.86 1.27,44.58 v2.03,43.81 2.03,42.55 2.41,42.16 4.06,42.16 4.29,41.94 LED4.4 | LED1.4 42.4,41.27 43.69,41.27 44.2,41.78 44.2,54.1 43.57,54.73 LED2.4 42.42,54.69 42.42,54.1 40.39,52.07 v40.01,52.07
  Bottom 0.406: v27.56,52.96 39.12,52.96 v40.01,52.07 | v1.91,40.39 3.56,38.73 v8.13,38.73 12.57,38.73 13.34,37.97 v13.34,35.05 13.34,35.18 13.97,35.81 20.32,35.81 21.59,34.54 v21.59,34.42 21.86,34.02 U$1.6 | v40.77,31.75 40.28,31.26 U$1.1 26.86,33.97 v26.67,34.42
VREG_IN
  Top 0.406: U$4.7 26.23,4.13 26.8,4.7 27.93,4.7 C2.1 28.02,4.76 U$9.P$1
VREG_OUT
  Top 0.254: S2.3 S2.2 35.83,62.09 39.12,58.8 43.56,58.8 44.45,57.91 44.45,20.95 38.61,15.11 38.61,2.16 37.85,1.4 30.48,1.4 29.91,1.96 U$9.P$3
VUSB
  Top 0.406: U2.VBUS1 10.13,4.22 10.54,3.81 14.86,3.81 18.41,7.37 F1.1

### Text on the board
tNames: https://hackaday.io/ / project/ / 26823-lameboy | ATTINY 13/45/85 | BC847S | BC847S | davedarko 2017 | SD | I2C | BC847S | + - | 12MHz | CH340G | TSP2113A | JST LIPO
bNames: ON | OFF | 84x48 DOT MATRIX DISPLAY | C | RST | G | LAMEBOY | V | D | C | A | B

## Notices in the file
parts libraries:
SparkFun-Connectors: Licensing: Creative Commons ShareAlike 4.0 International - https://creativecommons.org/licenses/by-sa/4.0
